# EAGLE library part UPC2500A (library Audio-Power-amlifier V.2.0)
45W AF power amplifier.
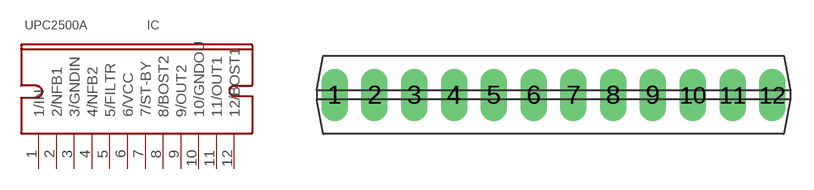
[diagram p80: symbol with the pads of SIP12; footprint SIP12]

Designator prefix IC

## UPC2500A  [SIP12]
1  1/IN  in
2  2/NFB1
3  3/GNDIN  pwr
4  4/NFB2
5  5/FILTR
6  6/VCC  pwr
7  7/ST-BY
8  8/BOST2
9  9/OUT2  out
10  10/GNDOU  pwr
11  11/OUT1  out
12  12/BOST1

## Footprint SIP12 (pad centres in mm)
drill 0.8 pad 1.676 long: 1 -13.97,0; 2 -11.43,0; 3 -8.89,0; 4 -6.35,0; 5 -3.81,0; 6 -1.27,0; 7 1.27,0; 8 3.81,0; 9 6.35,0; 10 8.89,0; 11 11.43,0; 12 13.97,0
